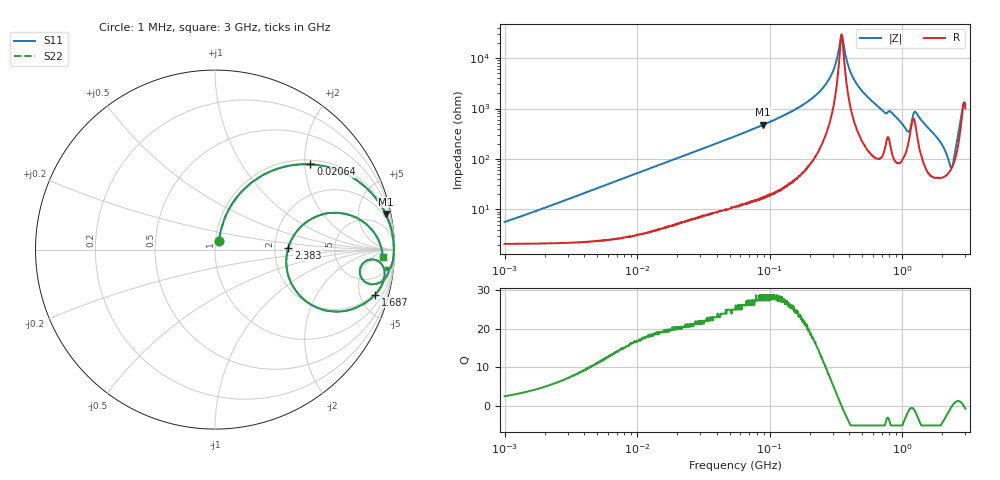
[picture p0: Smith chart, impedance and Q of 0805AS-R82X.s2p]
!s-Parameter Generated by FASTRON Sdn. Bhd.
!FASTRON P/N : 0805AS-R82X
!Keysight Technologies: E4991B_MY54100416_A.01.15
!Date: Mon Jun 15 12:56:13 2026
!Version  :Rev01  Mon Jun 15 12:56:13 2026
!Data & Calibration Information:
!Freq  S11  S21  S12  S22
!PortZ  Port1:50+j0  Port2:50+j0
!When reading reference impedance value at option line is always used.
! Remarks : This data is being provided solely for informational purposes.
# Hz S dB R 50
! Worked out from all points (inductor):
!   1601 points, 1 MHz to 3 GHz, reference 50 ohm
!   read as one part in series: L = 839 nH near 1.185 MHz
!   highest Q = 28.6 at 89.44 MHz (marker M1), where L = 846 nH
!   self-resonance near 348.9 MHz
!   S11 on the Smith chart (normalised r, x): 1 MHz: 1.04, +0.11; 20.64 MHz: 1.10, +2.13; 1.687 GHz: 1.89, -6.73; 2.383 GHz: 2.38, +0.07; 3 GHz: 21, -14
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1000000  -25.10 65.5  -0.19 -3.0  -0.19 -3.0  -25.10 65.5
3804036  -14.30 72.5  -0.36 -11.1  -0.36 -11.1  -14.30 72.5
1.447069e7  -4.62 51.1  -2.17 -35.9  -2.17 -35.9  -4.62 51.1
2.064365e7  -2.94 41.8  -3.52 -45.4  -3.52 -45.4  -2.94 41.8
5.504702e7  -0.61 19.1  -9.67 -68.6  -9.67 -68.6  -0.61 19.1
8.944052e7  -0.25 11.8  -13.80 -76.2  -13.80 -76.2  -0.25 11.8
2.083556e8  -0.05 3.6  -24.00 -83.2  -24.00 -83.2  -0.05 3.6
2.870054e8  -0.03 1.3  -32.60 -80.8  -32.60 -80.8  -0.03 1.3
3.10929e8  -0.03 0.8  -36.90 -75.8  -36.90 -75.8  -0.03 0.8
3.50605e8  -0.03 -0.0  -49.30 6.3  -49.30 6.3  -0.03 -0.0
3.973271e8  -0.03 -0.9  -36.00 75.7  -36.00 75.7  -0.03 -0.9
4.525341e8  -0.04 -1.8  -29.90 80.9  -29.90 80.9  -0.04 -1.8
7.135306e8  -0.17 -6.2  -19.30 76.3  -19.30 76.3  -0.17 -6.2
7.925923e8  -0.33 -6.0  -19.30 67.2  -19.30 67.2  -0.33 -6.0
1.097256e9  -1.33 -12.2  -12.30 48.3  -12.30 48.3  -1.33 -12.2
1.262285e9  -0.56 -5.4  -19.10 52.6  -19.10 52.6  -0.56 -5.4
1.687342e9  -0.66 -15.7  -11.30 66.8  -11.30 66.8  -0.66 -15.7
2.134733e9  -3.10 -28.9  -5.79 41.1  -5.79 41.1  -3.10 -28.9
2.383164e9  -7.77 1.6  -4.56 -1.1  -4.56 -1.1  -7.77 1.6
2.568929e9  -2.76 16.2  -8.79 -34.1  -8.79 -34.1  -2.76 16.2
2.853575e9  -0.74 2.4  -20.80 -24.5  -20.80 -24.5  -0.74 2.4
3e9  -0.57 -2.5  -22.30 32.1  -22.30 32.1  -0.57 -2.5
